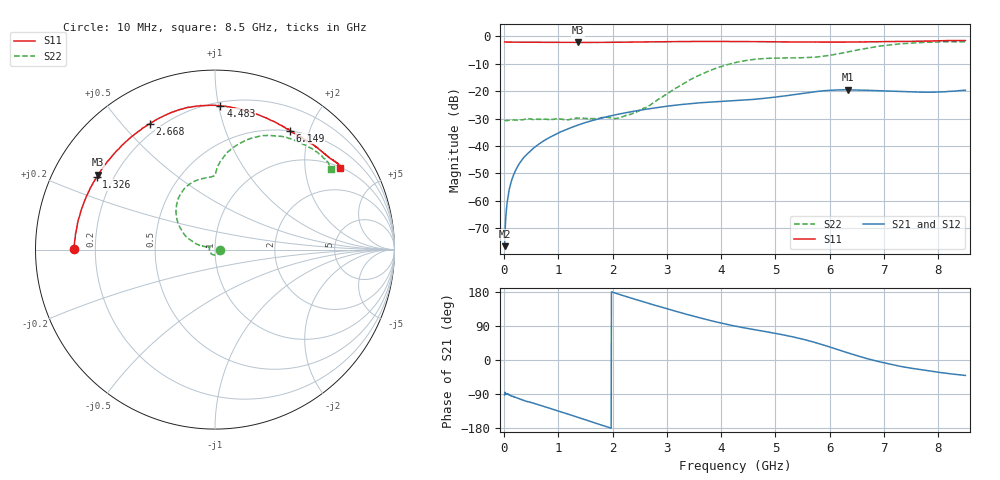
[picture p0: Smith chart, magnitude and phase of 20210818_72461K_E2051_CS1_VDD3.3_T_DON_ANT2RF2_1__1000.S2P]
!Agilent Technologies,E5071C,MY46417908,A.11.23
!Date: Wed Aug 18 14:26:11 2021
!Data & Calibration Information:
!Freq	S11:SOLT2(ON)	S21:SOLT2(ON)	S12:SOLT2(ON)	S22:SOLT2(ON)
!PortZ  Port1:50+j0  Port2:50+j0
!Above PortZ is port z conversion or system Z0 setting when saving the data.
!When reading, reference impedance value at option line is always used.
# Hz S dB R 50
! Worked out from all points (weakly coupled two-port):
!   1601 points, 10 MHz to 8.5 GHz, reference 50 ohm
!   highest |S21| = -19.49 dB at 6.34 GHz (marker M1); lowest = -76.5 dB at 10 MHz (marker M2)
!   lowest |S11| = -2.2 dB at 1.368 GHz (marker M3), VSWR 7.78, Z = 6.97 + j14.4 ohm
!   |S11| at or under -10 dB: nowhere
!   |S22| runs from -30.8 to -2.0 dB; largest |S21 - S12| = 0.00046
!   S11 on the Smith chart (normalised r, x): 10 MHz: 0.12, +0.00; 1.326 GHz: 0.14, +0.28; 2.668 GHz: 0.16, +0.60; 4.483 GHz: 0.23, +1.01; 6.149 GHz: 0.49, +1.70; 8.5 GHz: 1.01, +3.05
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1e7  -2.08 179.7  -76.51 -92.7  -76.19 -90.7  -30.50 -2.2
6.836875e7  -2.11 178.4  -58.85 -89.8  -58.87 -90.4  -30.69 -8.6
1.055125e8  -2.11 177.6  -54.94 -93.0  -54.99 -93.2  -30.58 -12.1
1.851062e8  -2.14 175.7  -50.11 -97.5  -50.04 -97.2  -30.46 -19.9
2.965375e8  -2.14 173.2  -45.94 -103.4  -45.98 -103.0  -30.55 -35.1
6.892e8  -2.19 163.9  -38.65 -120.6  -38.65 -120.5  -30.22 -87.1
1.32595e9  -2.23 148.4  -32.62 -149.7  -32.63 -149.6  -29.87 -165.1
1.3684e9  -2.24 147.3  -32.33 -151.6  -32.33 -151.6  -29.82 -168.7
1.426769e9  -2.23 145.8  -31.93 -154.4  -31.93 -154.3  -29.88 -173.6
2.100662e9  -2.16 129.1  -28.42 174.2  -28.42 174.2  -29.86 154.4
2.668431e9  -2.05 117.2  -26.43 149.3  -26.44 149.3  -25.37 163.1
2.843538e9  -2.00 114.1  -25.93 141.9  -25.94 141.8  -22.97 164.2
3.517431e9  -1.90 103.3  -24.40 114.7  -24.41 114.7  -14.94 155.4
4.255e9  -1.89 91.7  -23.46 89.6  -23.47 89.6  -9.62 130.2
4.483169e9  -1.92 87.8  -23.17 83.4  -23.18 83.5  -8.77 121.6
4.923588e9  -2.00 79.4  -22.35 72.2  -22.36 72.3  -8.00 105.8
5.671769e9  -2.10 65.2  -20.33 48.6  -20.33 48.7  -7.69 90.6
6.149331e9  -2.12 57.8  -19.56 27.4  -19.58 27.4  -6.43 87.3
6.340356e9  -2.08 55.2  -19.49 18.6  -19.52 18.6  -5.65 84.5
7.088538e9  -1.92 46.5  -19.95 -10.2  -19.98 -10.4  -3.17 66.3
7.911006e9  -1.67 37.5  -20.36 -30.4  -20.34 -30.4  -2.09 43.8
8.5e9  -1.57 33.2  -19.67 -40.8  -19.68 -41.0  -2.10 34.6
